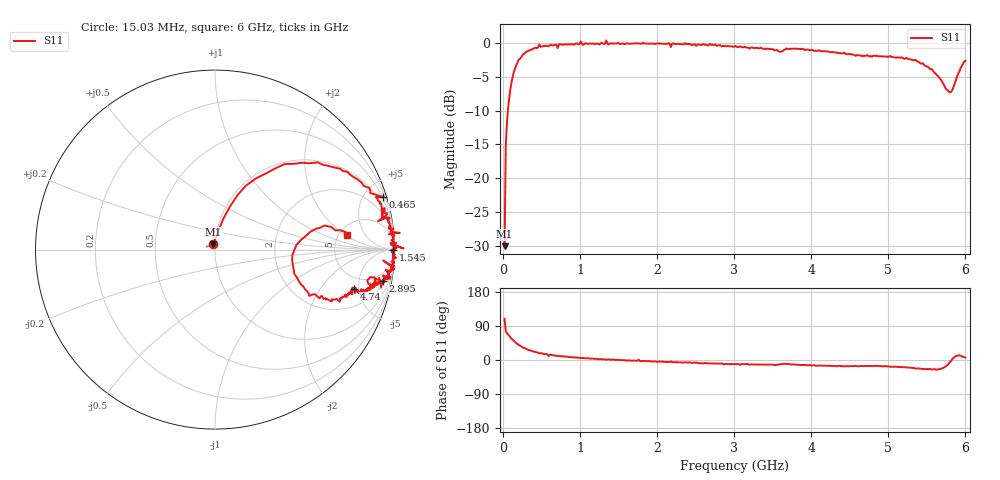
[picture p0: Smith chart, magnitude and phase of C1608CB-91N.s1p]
!	Network	Analyzer	HP8753E.07.74:	Oct	30	2002	Serial	No.	JP38451487
!	Hewlett-Packard
!	28	Aug	2009	8:27:52
!	Frequency	S11
#	HZ	S	RI	R	50
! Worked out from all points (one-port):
!   400 points, 15.03 MHz to 6 GHz, reference 50 ohm
!   lowest |S11| = -30.1 dB at 15.03 MHz (marker M1), VSWR 1.06, Z = 48.9 + j2.9 ohm
!   |S11| at or under -10 dB: start of sweep to 57.68 MHz
!   S11 on the Smith chart (normalised r, x): 15.03 MHz: 0.98, +0.06; 465 MHz: 0.40, +6.52; 1.545 GHz: open; 2.895 GHz: 3, -10; 4.74 GHz: 3.57, -4.46; 6 GHz: 5.84, +2.15
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1.502992e7  -0.0101 0.0296
3.002985e7  0.0449 0.169
6.00297e7  0.126 0.304
9.002955e7  0.229 0.397
1.350293e8  0.387 0.476
2.550287e8  0.698 0.45
4.650277e8  0.937 0.293
5.550272e8  0.919 0.266
5.850271e8  0.932 0.171
6.150269e8  0.946 0.231
7.650262e8  0.958 0.175
1.005025e9  1.03 0.0929
1.245024e9  0.978 0.0344
1.335023e9  1.05 0.00616
1.365023e9  0.98 0.0289
1.515022e9  0.985 -0.000793
1.545022e9  0.992 -9.16e-05
2.265019e9  0.987 -0.101
2.895016e9  0.935 -0.174
3.015015e9  0.941 -0.182
3.765011e9  0.893 -0.181
4.515007e9  0.8 -0.229
4.740006e9  0.776 -0.219
5.265004e9  0.718 -0.264
5.625002e9  0.525 -0.258
5.790001e9  0.43 -0.0622
5.895001e9  0.562 0.116
6e9  0.734 0.0837
